ORGANIZATION_BLOCK OB 1
BEGIN
	// Test DB1.DT1 initial values
	AUF DB 1
	LAR1		P#DBX 0.0
	L		B [AR1, P#0.0]
	__ASSERT==	__ACCU 1,	B#16#91
	L		B [AR1, P#1.0]
	__ASSERT==	__ACCU 1,	B#16#02
	L		B [AR1, P#2.0]
	__ASSERT==	__ACCU 1,	B#16#03
	L		B [AR1, P#3.0]
	__ASSERT==	__ACCU 1,	B#16#04
	L		B [AR1, P#4.0]
	__ASSERT==	__ACCU 1,	B#16#05
	L		B [AR1, P#5.0]
	__ASSERT==	__ACCU 1,	B#16#06
	L		B [AR1, P#6.0]
	__ASSERT==	__ACCU 1,	B#16#78
	L		B [AR1, P#7.0]
	__ASSERT==	__ACCU 1,	B#16#91

	// Test DB1.DT2 initial values
	AUF DB 1
	LAR1		P#DBX 8.0
	L		B [AR1, P#0.0]
	__ASSERT==	__ACCU 1,	B#16#10
	L		B [AR1, P#1.0]
	__ASSERT==	__ACCU 1,	B#16#11
	L		B [AR1, P#2.0]
	__ASSERT==	__ACCU 1,	B#16#12
	L		B [AR1, P#3.0]
	__ASSERT==	__ACCU 1,	B#16#13
	L		B [AR1, P#4.0]
	__ASSERT==	__ACCU 1,	B#16#14
	L		B [AR1, P#5.0]
	__ASSERT==	__ACCU 1,	B#16#15
	L		B [AR1, P#6.0]
	__ASSERT==	__ACCU 1,	B#16#16
	L		B [AR1, P#7.0]
	__ASSERT==	__ACCU 1,	B#16#06


	// Test DATE immediates
	L		D#1990-1-1
	__ASSERT==	__ACCU 1,	0
	L		DATE#1990-1-1
	__ASSERT==	__ACCU 1,	0
	L		D#2000-12-31
	__ASSERT==	__ACCU 1,	4017
	L		DATE#2000-12-31
	__ASSERT==	__ACCU 1,	4017
	L		D#2100-12-31
	__ASSERT==	__ACCU 1,	L#40541
	L		DATE#2100-12-31
	__ASSERT==	__ACCU 1,	L#40541
	L		D#2168-12-31
	__ASSERT==	__ACCU 1,	L#65378
	L		DATE#2168-12-31
	__ASSERT==	__ACCU 1,	L#65378
	// Test DB1.DATEx initial values
	L		DB1.DBW 16
	__ASSERT==	__ACCU 1,	4017
	L		DB1.DBW 18
	__ASSERT==	__ACCU 1,	L#40541


	// Test TIME_OF_DAY immediates
	L		TOD#0:0:0.0
	__ASSERT==	__ACCU 1,	0
	L		TIME_OF_DAY#0:0:0.0
	__ASSERT==	__ACCU 1,	0
	L		TOD#13:37:13.37
	__ASSERT==	__ACCU 1,	L#49033370
	L		TIME_OF_DAY#13:37:13.37
	__ASSERT==	__ACCU 1,	L#49033370
	L		TOD#23:59:59.999
	__ASSERT==	__ACCU 1,	L#86399999
	L		TIME_OF_DAY#23:59:59.999
	__ASSERT==	__ACCU 1,	L#86399999
	// Test DB1.TODx initial values
	L		DB1.DBD 20
	__ASSERT==	__ACCU 1,	L#86399999
	L		DB1.DBD 24
	__ASSERT==	__ACCU 1,	L#49033370


	// Test TIME immediates
	L		T#1s100ms
	__ASSERT==	__ACCU 1,	1100
	L		TIME#1s100ms
	__ASSERT==	__ACCU 1,	1100
	L		T#-1s100ms
	__ASSERT==	__ACCU 1,	L#-1100


	CALL SFC 46 // STOP CPU
END_ORGANIZATION_BLOCK


DATA_BLOCK DB 1
STRUCT
	DT1	: DATE_AND_TIME := DT#1990-1-1-0:0:0.0;
	DT2	: DATE_AND_TIME := DT#2010-11-12-13:14:15.16;
	DATE1	: DATE := D#2100-12-31;
	DATE2	: DATE := D#2100-12-31;
	TOD1	: TIME_OF_DAY := TOD#13:37:13.37;
	TOD2	: TIME_OF_DAY := TOD#13:37:13.37;
END_STRUCT;
BEGIN
	DT1	:= DATE_AND_TIME#1991-2-3-4:5:6.789;
	DATE1	:= D#2000-12-31;
	TOD1	:= TOD#23:59:59.999;
END_DATA_BLOCK
